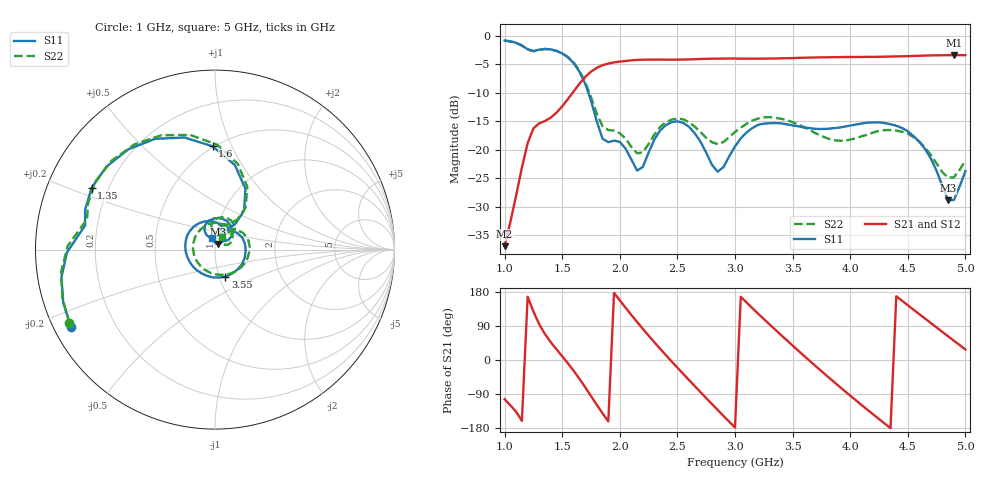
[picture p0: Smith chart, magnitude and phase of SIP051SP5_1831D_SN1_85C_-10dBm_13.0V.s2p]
# GHz  S  dB  R  50
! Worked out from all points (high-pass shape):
!   81 points, 1 GHz to 5 GHz, reference 50 ohm
!   highest |S21| = -3.38 dB at 4.9 GHz (marker M1); lowest = -36.9 dB at 1 GHz (marker M2)
!   |S21| within 3 dB of the highest: 1.744 GHz to end of sweep
!   lowest |S11| = -28.8 dB at 4.85 GHz (marker M3), VSWR 1.08, Z = 51.6 + j3.3 ohm
!   |S11| at or under -10 dB: 1.727 GHz to end of sweep
!   |S22| runs from -24.9 to -0.8 dB; largest |S21 - S12| = 0.0026
!   S11 on the Smith chart (normalised r, x): 1 GHz: 0.05, -0.25; 1.35 GHz: 0.14, +0.23; 1.6 GHz: 0.49, +0.85; 3.55 GHz: 1.07, -0.33; 5 GHz: 0.96, +0.12
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1  -0.81 -151.9  -36.88 -103.2  -37.08 -104.1  -0.83 -153.3
1.2  -2.35 173.8  -18.83 166.9  -18.85 166.9  -2.40 171.0
1.35  -2.29 153.4  -14.94 68.5  -14.90 68.4  -2.31 150.3
1.6  -4.80 91.3  -9.73 -28.6  -9.72 -28.7  -4.67 88.7
1.7  -8.43 63.4  -7.21 -72.1  -7.22 -72.0  -8.12 62.7
1.8  -14.98 51.5  -5.61 -118.2  -5.59 -118.1  -13.64 53.3
1.95  -18.37 80.8  -4.66 177.2  -4.66 177.2  -16.62 71.5
2.15  -23.62 91.5  -4.22 100.5  -4.22 100.5  -20.61 79.1
2.35  -16.60 111.5  -4.16 29.7  -4.15 29.7  -15.96 94.2
2.5  -14.99 78.9  -4.17 -20.2  -4.16 -20.2  -14.52 69.3
2.7  -18.53 39.1  -4.05 -84.6  -4.05 -84.6  -16.88 43.0
2.85  -23.82 52.2  -4.00 -132.0  -3.98 -132.0  -18.98 48.2
3  -19.40 65.1  -3.98 -178.2  -3.96 -178.2  -16.86 50.0
3.3  -15.33 -1.5  -3.98 94.0  -3.98 93.9  -14.25 5.3
3.55  -15.87 -69.1  -3.86 24.4  -3.85 24.4  -15.55 -46.7
3.7  -16.32 -107.5  -3.79 -16.1  -3.79 -16.0  -17.09 -85.3
4  -15.73 -175.6  -3.71 -93.9  -3.71 -94.0  -18.20 177.1
4.35  -15.50 111.5  -3.63 -179.9  -3.64 -179.9  -16.52 81.6
4.6  -18.57 63.1  -3.50 121.0  -3.49 120.9  -18.56 34.0
4.85  -28.82 61.9  -3.38 62.5  -3.38 62.5  -24.88 33.9
4.9  -28.79 85.1  -3.38 50.9  -3.38 50.9  -24.80 47.4
5  -23.74 105.3  -3.39 27.9  -3.38 27.8  -21.86 61.6
